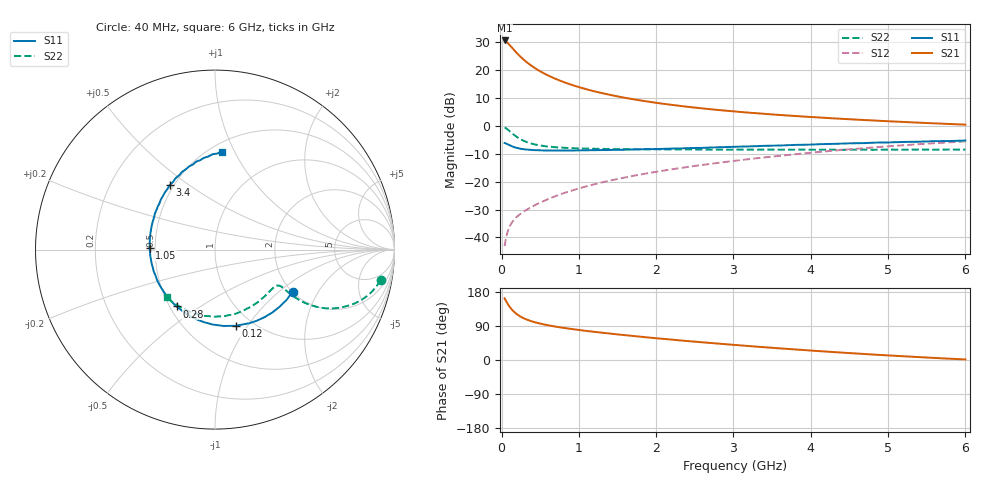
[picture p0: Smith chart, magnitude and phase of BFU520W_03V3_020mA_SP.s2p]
! Filename:  P:\Prog\Test\Noise\ATS_data\Testdata_Net\Run2\BFU520W_APM2013_06_A05_03p3V_020mA_SP_CM01_D.s2p
! Date/Time: Tue 26/Mar/2013 18:01:39
! BFU520W_APM2013_06_A05_03p3V_1to20mA_SP_CM01_Bias8_R.s2p
! MDIF S-parameter v. bias file
! BFU520W_APM2013_06_A05_03p3V_1to20mA_SP_CM01
! Date/time Tue Mar 19 16:47:37 2013
! VAR V_out= 3.3000
! VAR I_out= 20.0000
! VAR V_in= 0.8605
! VAR I_in= 0.2417
! Device data file deembeded for feedlines and parallel
! Original file: \Run2\BFU520W_APM2013_06_A05_03p3V_020mA_SP_CM01_R.s2p
! Feed-files: PR019V01_070313_Feed1.s2p, PR019V01_070313_Feed2.s2p
! Parallel-file: PR019V01_070313_Par.s2p
# MHz S MA R 50
!  Freq-MHz  S11-mag  S11-arg  S21-mag  S21-arg  S12-mag  S12-arg  S22-mag  S22-arg
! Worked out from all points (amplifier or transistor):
!   98 points, 40 MHz to 6 GHz, reference 50 ohm
!   highest |S21| = 30.6 dB at 40 MHz (marker M1)
!   |S21| within 3 dB of that: start of sweep to 148.7 MHz
!   unconditionally stable (mu >= 1): 780.4 MHz to 1.989 GHz
!   at 300 MHz: K = 0.74, MSG = 27.0 dB, |S12| = -30.5 dB
!   at 1.6 GHz: K = 1.02, MAG = 13.4 dB, |S12| = -18.5 dB
!   at 6 GHz: K = 0.82, MSG = 3.0 dB, |S12| = -5.6 dB
!   S11 on the Smith chart (normalised r, x): 40 MHz: 2.01, -1.24; 120 MHz: 0.84, -0.88; 280 MHz: 0.54, -0.40; 1.05 GHz: 0.47, +0.01; 3.4 GHz: 0.48, +0.42; 6 GHz: 0.57, +0.89
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40  0.492 -28.6  33.94 162.7  0.006971 79.7  0.9392 -10.5
50  0.4874 -35.2  33.43 158.8  0.008537 77.8  0.922 -12.9
60  0.4802 -41.9  32.28 155.0  0.01004 75.7  0.9033 -15.2
80  0.4665 -54.0  30.5 148.1  0.01275 72.2  0.8603 -19.2
100  0.4528 -64.9  28.55 141.9  0.01512 69.5  0.8145 -22.3
120  0.4397 -74.9  26.67 136.4  0.01717 67.3  0.7706 -24.8
160  0.4178 -91.5  23.05 127.6  0.02064 64.6  0.6927 -28.1
200  0.402 -104.7  20.07 120.8  0.02354 63.5  0.6303 -29.9
240  0.3901 -115.3  17.66 115.3  0.02612 63.4  0.5823 -30.6
280  0.382 -124.0  15.69 110.9  0.02861 63.7  0.5453 -30.9
340  0.3747 -134.2  13.37 105.7  0.03223 64.7  0.5047 -30.7
400  0.3687 -142.2  11.62 101.5  0.03589 65.9  0.4762 -30.3
550  0.3615 -156.7  8.709 93.8  0.04518 68.8  0.4339 -29.3
750  0.3614 -168.9  6.512 86.4  0.05836 71.3  0.4093 -29.3
1050  0.3637 178.3  4.731 78.0  0.07902 73.3  0.393 -31.4
1500  0.3718 164.5  3.377 67.5  0.1115 73.8  0.3836 -37.1
2050  0.3854 151.3  2.531 56.5  0.1538 72.6  0.379 -45.7
3100  0.4252 130.4  1.77 38.4  0.2439 67.2  0.3757 -65.7
3400  0.4387 125.3  1.642 33.8  0.2718 65.0  0.3752 -72.2
4100  0.468 113.6  1.415 23.6  0.3398 59.2  0.3726 -87.7
5200  0.5147 97.0  1.175 9.8  0.4496 48.2  0.373 -114.4
6000  0.5459 86.0  1.051 1.5  0.5247 39.3  0.3745 -135.4
